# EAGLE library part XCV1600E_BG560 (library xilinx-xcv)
xcv1600e_bg560 edit this description Auto generated by make-symbol-device-package-bsdl.ulp Rev. 26 Source: xcv1600e_bg560.bsd
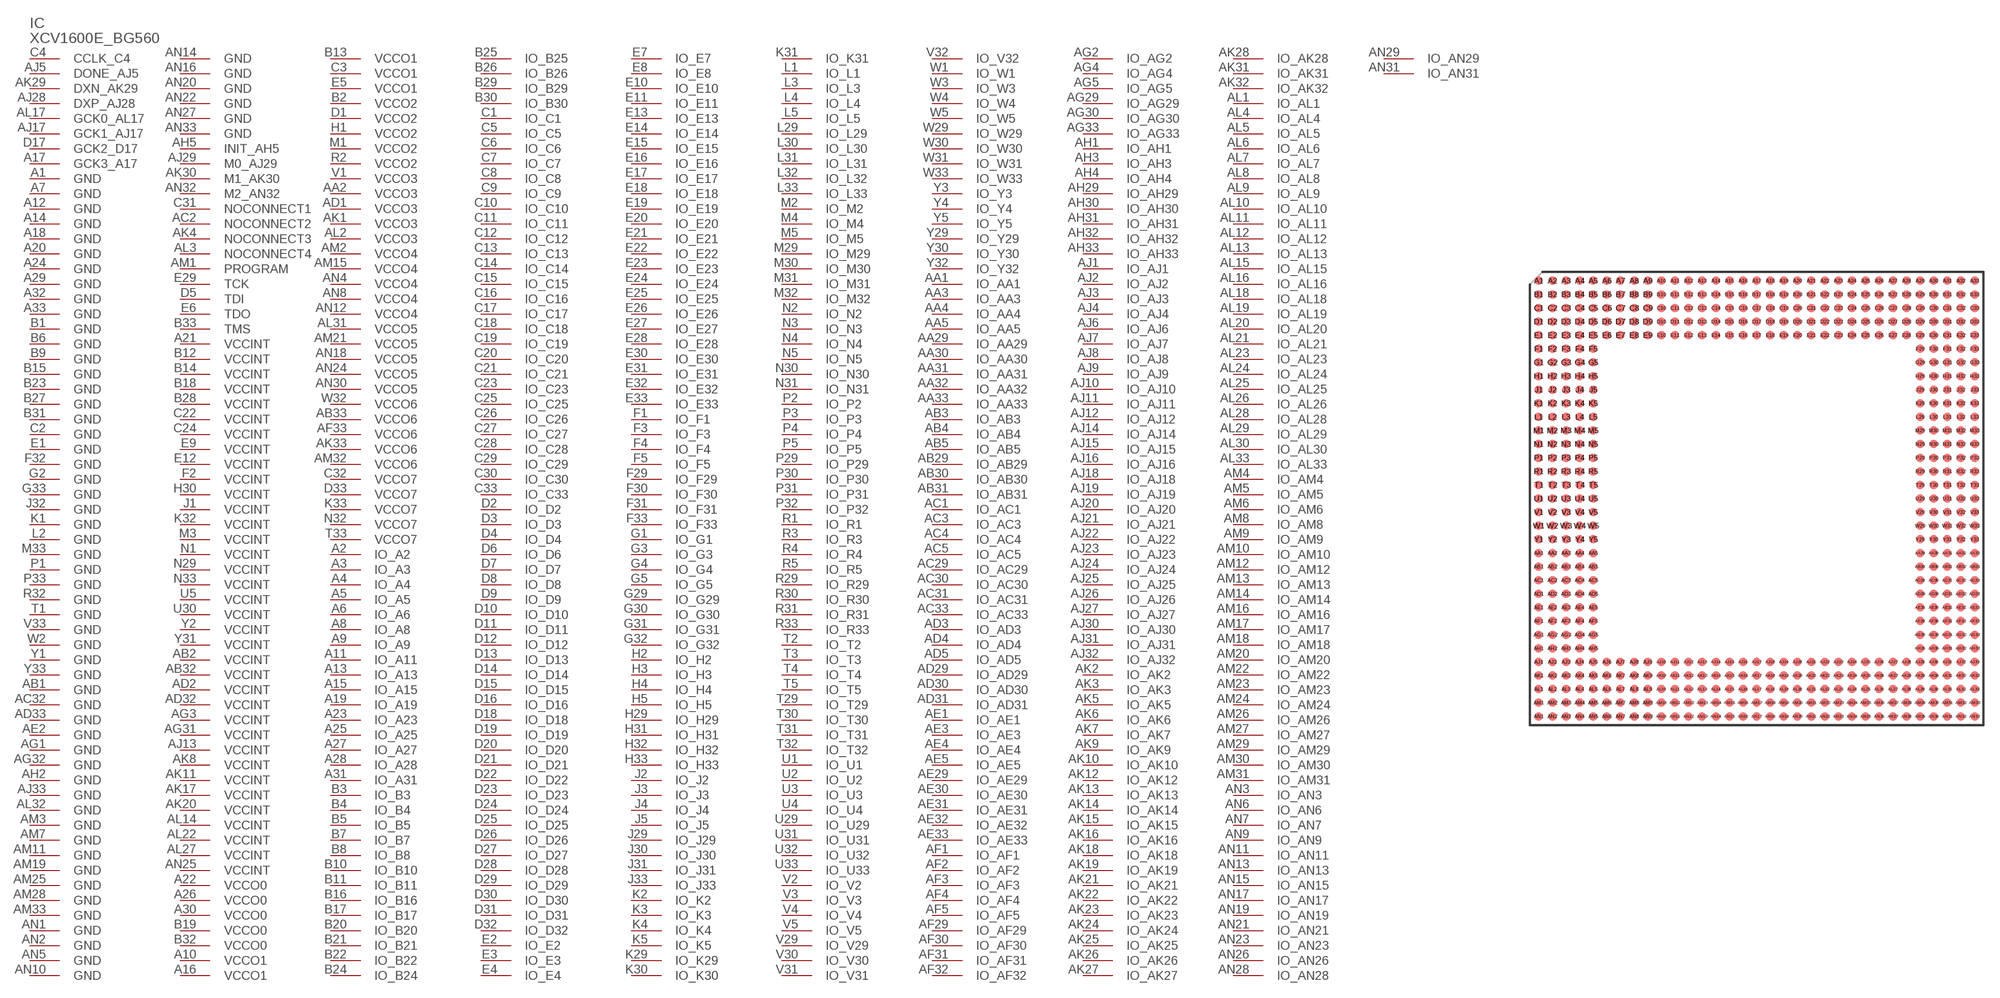
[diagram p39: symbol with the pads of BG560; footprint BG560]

Designator prefix IC

## XCV1600E_BG560 (OC_FARNELL: unknown; OC_NEWARK: unknown)  [BG560]
A1  GND  pwr
A2  IO_A2
A3  IO_A3
A4  IO_A4
A5  IO_A5
A6  IO_A6
A7  GND  pwr
A8  IO_A8
A9  IO_A9
A10  VCCO1  pwr
A11  IO_A11
A12  GND  pwr
A13  IO_A13
A14  GND  pwr
A15  IO_A15
A16  VCCO1  pwr
A17  GCK3_A17  in
A18  GND  pwr
A19  IO_A19
A20  GND  pwr
A21  VCCINT  pwr
A22  VCCO0  pwr
A23  IO_A23
A24  GND  pwr
A25  IO_A25
A26  VCCO0  pwr
A27  IO_A27
A28  IO_A28
A29  GND  pwr
A30  VCCO0  pwr
A31  IO_A31
A32  GND  pwr
A33  GND  pwr
AA1  IO_AA1
AA2  VCCO3  pwr
AA3  IO_AA3
AA4  IO_AA4
AA5  IO_AA5
AA29  IO_AA29
AA30  IO_AA30
AA31  IO_AA31
AA32  IO_AA32
AA33  IO_AA33
AB1  GND  pwr
AB2  VCCINT  pwr
AB3  IO_AB3
AB4  IO_AB4
AB5  IO_AB5
AB29  IO_AB29
AB30  IO_AB30
AB31  IO_AB31
AB32  VCCINT  pwr
AB33  VCCO6  pwr
AC1  IO_AC1
AC2  NOCONNECT2  pas
AC3  IO_AC3
AC4  IO_AC4
AC5  IO_AC5
AC29  IO_AC29
AC30  IO_AC30
AC31  IO_AC31
AC32  GND  pwr
AC33  IO_AC33
AD1  VCCO3  pwr
AD2  VCCINT  pwr
AD3  IO_AD3
AD4  IO_AD4
AD5  IO_AD5
AD29  IO_AD29
AD30  IO_AD30
AD31  IO_AD31
AD32  VCCINT  pwr
AD33  GND  pwr
AE1  IO_AE1
AE2  GND  pwr
AE3  IO_AE3
AE4  IO_AE4
AE5  IO_AE5
AE29  IO_AE29
AE30  IO_AE30
AE31  IO_AE31
AE32  IO_AE32
AE33  IO_AE33
AF1  IO_AF1
AF2  IO_AF2
AF3  IO_AF3
AF4  IO_AF4
AF5  IO_AF5
AF29  IO_AF29
AF30  IO_AF30
AF31  IO_AF31
AF32  IO_AF32
AF33  VCCO6  pwr
AG1  GND  pwr
AG2  IO_AG2
AG3  VCCINT  pwr
AG4  IO_AG4
AG5  IO_AG5
AG29  IO_AG29
AG30  IO_AG30
AG31  VCCINT  pwr
AG32  GND  pwr
AG33  IO_AG33
AH1  IO_AH1
AH2  GND  pwr
AH3  IO_AH3
AH4  IO_AH4
AH5  INIT_AH5
AH29  IO_AH29
AH30  IO_AH30
AH31  IO_AH31
AH32  IO_AH32
AH33  IO_AH33
AJ1  IO_AJ1
AJ2  IO_AJ2
AJ3  IO_AJ3
AJ4  IO_AJ4
AJ5  DONE_AJ5
AJ6  IO_AJ6
AJ7  IO_AJ7
AJ8  IO_AJ8
AJ9  IO_AJ9
AJ10  IO_AJ10
AJ11  IO_AJ11
AJ12  IO_AJ12
AJ13  VCCINT  pwr
AJ14  IO_AJ14
AJ15  IO_AJ15
AJ16  IO_AJ16
AJ17  GCK1_AJ17  in
AJ18  IO_AJ18
AJ19  IO_AJ19
AJ20  IO_AJ20
AJ21  IO_AJ21
AJ22  IO_AJ22
AJ23  IO_AJ23
AJ24  IO_AJ24
AJ25  IO_AJ25
AJ26  IO_AJ26
AJ27  IO_AJ27
AJ28  DXP_AJ28  pas
AJ29  M0_AJ29  in
AJ30  IO_AJ30
AJ31  IO_AJ31
AJ32  IO_AJ32
AJ33  GND  pwr
AK1  VCCO3  pwr
AK2  IO_AK2
AK3  IO_AK3
AK4  NOCONNECT3  pas
AK5  IO_AK5
AK6  IO_AK6
AK7  IO_AK7
AK8  VCCINT  pwr
AK9  IO_AK9
AK10  IO_AK10
AK11  VCCINT  pwr
AK12  IO_AK12
AK13  IO_AK13
AK14  IO_AK14
AK15  IO_AK15
AK16  IO_AK16
AK17  VCCINT  pwr
AK18  IO_AK18
AK19  IO_AK19
AK20  VCCINT  pwr
AK21  IO_AK21
AK22  IO_AK22
AK23  IO_AK23
AK24  IO_AK24
AK25  IO_AK25
AK26  IO_AK26
AK27  IO_AK27
AK28  IO_AK28
AK29  DXN_AK29  pas
AK30  M1_AK30  in
AK31  IO_AK31
AK32  IO_AK32
AK33  VCCO6  pwr
AL1  IO_AL1
AL2  VCCO3  pwr
AL3  NOCONNECT4  pas
AL4  IO_AL4
AL5  IO_AL5
AL6  IO_AL6
AL7  IO_AL7
AL8  IO_AL8
AL9  IO_AL9
AL10  IO_AL10
AL11  IO_AL11
AL12  IO_AL12
AL13  IO_AL13
AL14  VCCINT  pwr
AL15  IO_AL15
AL16  IO_AL16
AL17  GCK0_AL17  in
AL18  IO_AL18
AL19  IO_AL19
AL20  IO_AL20
AL21  IO_AL21
AL22  VCCINT  pwr
AL23  IO_AL23
AL24  IO_AL24
AL25  IO_AL25
AL26  IO_AL26
AL27  VCCINT  pwr
AL28  IO_AL28
AL29  IO_AL29
AL30  IO_AL30
AL31  VCCO5  pwr
AL32  GND  pwr
AL33  IO_AL33
AM1  PROGRAM  in
AM2  VCCO4  pwr
AM3  GND  pwr
AM4  IO_AM4
AM5  IO_AM5
AM6  IO_AM6
AM7  GND  pwr
AM8  IO_AM8
AM9  IO_AM9
AM10  IO_AM10
AM11  GND  pwr
AM12  IO_AM12
AM13  IO_AM13
AM14  IO_AM14
AM15  VCCO4  pwr
AM16  IO_AM16
AM17  IO_AM17
AM18  IO_AM18
AM19  GND  pwr
AM20  IO_AM20
AM21  VCCO5  pwr
AM22  IO_AM22
AM23  IO_AM23
AM24  IO_AM24
AM25  GND  pwr
AM26  IO_AM26
AM27  IO_AM27
AM28  GND  pwr
AM29  IO_AM29
AM30  IO_AM30
AM31  IO_AM31
AM32  VCCO6  pwr
AM33  GND  pwr
AN1  GND  pwr
AN2  GND  pwr
AN3  IO_AN3
AN4  VCCO4  pwr
AN5  GND  pwr
AN6  IO_AN6
AN7  IO_AN7
AN8  VCCO4  pwr
AN9  IO_AN9
AN10  GND  pwr
AN11  IO_AN11
AN12  VCCO4  pwr
AN13  IO_AN13
AN14  GND  pwr
AN15  IO_AN15
AN16  GND  pwr
AN17  IO_AN17
AN18  VCCO5  pwr
AN19  IO_AN19
AN20  GND  pwr
AN21  IO_AN21
AN22  GND  pwr
AN23  IO_AN23
AN24  VCCO5  pwr
AN25  VCCINT  pwr
AN26  IO_AN26
AN27  GND  pwr
AN28  IO_AN28
AN29  IO_AN29
AN30  VCCO5  pwr
AN31  IO_AN31
AN32  M2_AN32  in
AN33  GND  pwr
B1  GND  pwr
B2  VCCO2  pwr
B3  IO_B3
B4  IO_B4
B5  IO_B5
B6  GND  pwr
B7  IO_B7
B8  IO_B8
B9  GND  pwr
B10  IO_B10
B11  IO_B11
B12  VCCINT  pwr
B13  VCCO1  pwr
B14  VCCINT  pwr
B15  GND  pwr
B16  IO_B16
B17  IO_B17
B18  VCCINT  pwr
B19  VCCO0  pwr
B20  IO_B20
B21  IO_B21
B22  IO_B22
B23  GND  pwr
B24  IO_B24
B25  IO_B25
B26  IO_B26
B27  GND  pwr
B28  VCCINT  pwr
B29  IO_B29
B30  IO_B30
B31  GND  pwr
B32  VCCO0  pwr
B33  TMS  in
C1  IO_C1
C2  GND  pwr
C3  VCCO1  pwr
C4  CCLK_C4
C5  IO_C5
C6  IO_C6
C7  IO_C7
C8  IO_C8
C9  IO_C9
C10  IO_C10
C11  IO_C11
C12  IO_C12
C13  IO_C13
C14  IO_C14
C15  IO_C15
C16  IO_C16
C17  IO_C17
C18  IO_C18
C19  IO_C19
C20  IO_C20
C21  IO_C21
C22  VCCINT  pwr
C23  IO_C23
C24  VCCINT  pwr
C25  IO_C25
C26  IO_C26
C27  IO_C27
C28  IO_C28
C29  IO_C29
C30  IO_C30
C31  NOCONNECT1  pas
C32  VCCO7  pwr
C33  IO_C33
D1  VCCO2  pwr
D2  IO_D2
D3  IO_D3
D4  IO_D4
D5  TDI  in
D6  IO_D6
D7  IO_D7
D8  IO_D8
D9  IO_D9
D10  IO_D10
D11  IO_D11
D12  IO_D12
D13  IO_D13
D14  IO_D14
D15  IO_D15
D16  IO_D16
D17  GCK2_D17  in
D18  IO_D18
D19  IO_D19
D20  IO_D20
D21  IO_D21
D22  IO_D22
D23  IO_D23
D24  IO_D24
D25  IO_D25
D26  IO_D26
D27  IO_D27
D28  IO_D28
D29  IO_D29
D30  IO_D30
D31  IO_D31
D32  IO_D32
D33  VCCO7  pwr
E1  GND  pwr
E2  IO_E2
E3  IO_E3
E4  IO_E4
E5  VCCO1  pwr
E6  TDO  out
E7  IO_E7
E8  IO_E8
E9  VCCINT  pwr
E10  IO_E10
E11  IO_E11
E12  VCCINT  pwr
E13  IO_E13
E14  IO_E14
E15  IO_E15
E16  IO_E16
E17  IO_E17
E18  IO_E18
E19  IO_E19
E20  IO_E20
E21  IO_E21
E22  IO_E22
E23  IO_E23
E24  IO_E24
E25  IO_E25
E26  IO_E26
E27  IO_E27
E28  IO_E28
E29  TCK  in
E30  IO_E30
E31  IO_E31
E32  IO_E32
E33  IO_E33
F1  IO_F1
F2  VCCINT  pwr
F3  IO_F3
F4  IO_F4
F5  IO_F5
F29  IO_F29
F30  IO_F30
F31  IO_F31
F32  GND  pwr
F33  IO_F33
G1  IO_G1
G2  GND  pwr
G3  IO_G3
G4  IO_G4
G5  IO_G5
G29  IO_G29
G30  IO_G30
G31  IO_G31
G32  IO_G32
G33  GND  pwr
H1  VCCO2  pwr
H2  IO_H2
H3  IO_H3
H4  IO_H4
H5  IO_H5
H29  IO_H29
H30  VCCINT  pwr
H31  IO_H31
H32  IO_H32
H33  IO_H33
J1  VCCINT  pwr
J2  IO_J2
J3  IO_J3
J4  IO_J4
J5  IO_J5
J29  IO_J29
J30  IO_J30
J31  IO_J31
J32  GND  pwr
J33  IO_J33
K1  GND  pwr
K2  IO_K2
K3  IO_K3
K4  IO_K4
K5  IO_K5
K29  IO_K29
K30  IO_K30
K31  IO_K31
K32  VCCINT  pwr
K33  VCCO7  pwr
L1  IO_L1
L2  GND  pwr
L3  IO_L3
L4  IO_L4
L5  IO_L5
L29  IO_L29
L30  IO_L30
L31  IO_L31
L32  IO_L32
L33  IO_L33
M1  VCCO2  pwr
M2  IO_M2
M3  VCCINT  pwr
M4  IO_M4
M5  IO_M5
M29  IO_M29
M30  IO_M30
M31  IO_M31
M32  IO_M32
M33  GND  pwr
N1  VCCINT  pwr
N2  IO_N2
N3  IO_N3
N4  IO_N4
N5  IO_N5
N29  VCCINT  pwr
N30  IO_N30
N31  IO_N31
N32  VCCO7  pwr
N33  VCCINT  pwr
P1  GND  pwr
P2  IO_P2
P3  IO_P3
P4  IO_P4
P5  IO_P5
P29  IO_P29
P30  IO_P30
P31  IO_P31
P32  IO_P32
P33  GND  pwr
R1  IO_R1
R2  VCCO2  pwr
R3  IO_R3
R4  IO_R4
R5  IO_R5
R29  IO_R29
R30  IO_R30
R31  IO_R31
R32  GND  pwr
R33  IO_R33
T1  GND  pwr
T2  IO_T2
T3  IO_T3
T4  IO_T4
T5  IO_T5
T29  IO_T29
T30  IO_T30
T31  IO_T31
T32  IO_T32
T33  VCCO7  pwr
U1  IO_U1
U2  IO_U2
U3  IO_U3
U4  IO_U4
U5  VCCINT  pwr
U29  IO_U29
U30  VCCINT  pwr
U31  IO_U31
U32  IO_U32
U33  IO_U33
V1  VCCO3  pwr
V2  IO_V2
V3  IO_V3
V4  IO_V4
V5  IO_V5
V29  IO_V29
V30  IO_V30
V31  IO_V31
V32  IO_V32
V33  GND  pwr
W1  IO_W1
W2  GND  pwr
W3  IO_W3
W4  IO_W4
W5  IO_W5
W29  IO_W29
W30  IO_W30
W31  IO_W31
W32  VCCO6  pwr
W33  IO_W33
Y1  GND  pwr
Y2  VCCINT  pwr
Y3  IO_Y3
Y4  IO_Y4
Y5  IO_Y5
Y29  IO_Y29
Y30  IO_Y30
Y31  VCCINT  pwr
Y32  IO_Y32
Y33  GND  pwr

## Footprint BG560 (pad centres in mm)
Metal BGA (BG560) Auto generated by make-symbol-device-package-bsdl.ulp Rev. 26 Source: xcv1000_bg560_1532.bsd; bg560.pdf
smd 0.8 x 0.8: A1 -20.32,20.32; A2 -19.05,20.32; A3 -17.78,20.32; A4 -16.51,20.32; A5 -15.24,20.32; A6 -13.97,20.32; A7 -12.7,20.32; A8 -11.43,20.32; A9 -10.16,20.32; A10 -8.89,20.32; A11 -7.62,20.32; A12 -6.35,20.32; A13 -5.08,20.32; A14 -3.81,20.32; A15 -2.54,20.32; A16 -1.27,20.32; A17 0,20.32; A18 1.27,20.32; A19 2.54,20.32; A20 3.81,20.32; A21 5.08,20.32; A22 6.35,20.32; A23 7.62,20.32; A24 8.89,20.32; A25 10.16,20.32; A26 11.43,20.32; A27 12.7,20.32; A28 13.97,20.32; A29 15.24,20.32; A30 16.51,20.32; A31 17.78,20.32; A32 19.05,20.32; A33 20.32,20.32; AA1 -20.32,-5.08; AA2 -19.05,-5.08; AA3 -17.78,-5.08; AA4 -16.51,-5.08; AA5 -15.24,-5.08; AA29 15.24,-5.08; AA30 16.51,-5.08; AA31 17.78,-5.08; AA32 19.05,-5.08; AA33 20.32,-5.08; AB1 -20.32,-6.35; AB2 -19.05,-6.35; AB3 -17.78,-6.35; AB4 -16.51,-6.35; AB5 -15.24,-6.35; AB29 15.24,-6.35; AB30 16.51,-6.35; AB31 17.78,-6.35; AB32 19.05,-6.35; AB33 20.32,-6.35; AC1 -20.32,-7.62; AC2 -19.05,-7.62; AC3 -17.78,-7.62; AC4 -16.51,-7.62; AC5 -15.24,-7.62; AC29 15.24,-7.62; AC30 16.51,-7.62; AC31 17.78,-7.62; AC32 19.05,-7.62; AC33 20.32,-7.62; AD1 -20.32,-8.89; AD2 -19.05,-8.89; AD3 -17.78,-8.89; AD4 -16.51,-8.89; AD5 -15.24,-8.89; AD29 15.24,-8.89; AD30 16.51,-8.89; AD31 17.78,-8.89; AD32 19.05,-8.89; AD33 20.32,-8.89; AE1 -20.32,-10.16; AE2 -19.05,-10.16; AE3 -17.78,-10.16; AE4 -16.51,-10.16; AE5 -15.24,-10.16; AE29 15.24,-10.16; AE30 16.51,-10.16; AE31 17.78,-10.16; AE32 19.05,-10.16; AE33 20.32,-10.16; AF1 -20.32,-11.43; AF2 -19.05,-11.43; AF3 -17.78,-11.43; AF4 -16.51,-11.43; AF5 -15.24,-11.43; AF29 15.24,-11.43; AF30 16.51,-11.43; AF31 17.78,-11.43; AF32 19.05,-11.43; AF33 20.32,-11.43; AG1 -20.32,-12.7; AG2 -19.05,-12.7; AG3 -17.78,-12.7; AG4 -16.51,-12.7; AG5 -15.24,-12.7; AG29 15.24,-12.7; AG30 16.51,-12.7; AG31 17.78,-12.7; AG32 19.05,-12.7; AG33 20.32,-12.7; AH1 -20.32,-13.97; AH2 -19.05,-13.97; AH3 -17.78,-13.97; AH4 -16.51,-13.97; AH5 -15.24,-13.97; AH29 15.24,-13.97; AH30 16.51,-13.97; AH31 17.78,-13.97; AH32 19.05,-13.97; AH33 20.32,-13.97; AJ1 -20.32,-15.24; AJ2 -19.05,-15.24; AJ3 -17.78,-15.24; AJ4 -16.51,-15.24; AJ5 -15.24,-15.24; AJ6 -13.97,-15.24; AJ7 -12.7,-15.24; AJ8 -11.43,-15.24; AJ9 -10.16,-15.24; AJ10 -8.89,-15.24; AJ11 -7.62,-15.24; AJ12 -6.35,-15.24; AJ13 -5.08,-15.24; AJ14 -3.81,-15.24; AJ15 -2.54,-15.24; AJ16 -1.27,-15.24; AJ17 0,-15.24; AJ18 1.27,-15.24; AJ19 2.54,-15.24; AJ20 3.81,-15.24; AJ21 5.08,-15.24; AJ22 6.35,-15.24; AJ23 7.62,-15.24; AJ24 8.89,-15.24; AJ25 10.16,-15.24; AJ26 11.43,-15.24; AJ27 12.7,-15.24; AJ28 13.97,-15.24; AJ29 15.24,-15.24; AJ30 16.51,-15.24; AJ31 17.78,-15.24; AJ32 19.05,-15.24; AJ33 20.32,-15.24; AK1 -20.32,-16.51; AK2 -19.05,-16.51; AK3 -17.78,-16.51; AK4 -16.51,-16.51; AK5 -15.24,-16.51; AK6 -13.97,-16.51; AK7 -12.7,-16.51; AK8 -11.43,-16.51; AK9 -10.16,-16.51; AK10 -8.89,-16.51; AK11 -7.62,-16.51; AK12 -6.35,-16.51; AK13 -5.08,-16.51; AK14 -3.81,-16.51; AK15 -2.54,-16.51; AK16 -1.27,-16.51; AK17 0,-16.51; AK18 1.27,-16.51; AK19 2.54,-16.51; AK20 3.81,-16.51; AK21 5.08,-16.51; AK22 6.35,-16.51; AK23 7.62,-16.51; AK24 8.89,-16.51; AK25 10.16,-16.51; AK26 11.43,-16.51; AK27 12.7,-16.51; AK28 13.97,-16.51; AK29 15.24,-16.51; AK30 16.51,-16.51; AK31 17.78,-16.51; AK32 19.05,-16.51; AK33 20.32,-16.51; AL1 -20.32,-17.78; AL2 -19.05,-17.78; AL3 -17.78,-17.78; AL4 -16.51,-17.78; AL5 -15.24,-17.78; AL6 -13.97,-17.78; AL7 -12.7,-17.78; AL8 -11.43,-17.78; AL9 -10.16,-17.78; AL10 -8.89,-17.78; AL11 -7.62,-17.78; AL12 -6.35,-17.78; AL13 -5.08,-17.78; AL14 -3.81,-17.78; AL15 -2.54,-17.78; AL16 -1.27,-17.78; AL17 0,-17.78; AL18 1.27,-17.78; AL19 2.54,-17.78; AL20 3.81,-17.78; AL21 5.08,-17.78; AL22 6.35,-17.78; AL23 7.62,-17.78; AL24 8.89,-17.78; AL25 10.16,-17.78; AL26 11.43,-17.78; AL27 12.7,-17.78; AL28 13.97,-17.78; AL29 15.24,-17.78; AL30 16.51,-17.78; AL31 17.78,-17.78; AL32 19.05,-17.78; AL33 20.32,-17.78; AM1 -20.32,-19.05; AM2 -19.05,-19.05; AM3 -17.78,-19.05; AM4 -16.51,-19.05; AM5 -15.24,-19.05; AM6 -13.97,-19.05; AM7 -12.7,-19.05; AM8 -11.43,-19.05; AM9 -10.16,-19.05; AM10 -8.89,-19.05; AM11 -7.62,-19.05; AM12 -6.35,-19.05; AM13 -5.08,-19.05; AM14 -3.81,-19.05; AM15 -2.54,-19.05; AM16 -1.27,-19.05; AM17 0,-19.05; AM18 1.27,-19.05; AM19 2.54,-19.05; AM20 3.81,-19.05; AM21 5.08,-19.05; AM22 6.35,-19.05; AM23 7.62,-19.05; AM24 8.89,-19.05; AM25 10.16,-19.05; AM26 11.43,-19.05; AM27 12.7,-19.05; AM28 13.97,-19.05; AM29 15.24,-19.05; AM30 16.51,-19.05; AM31 17.78,-19.05; AM32 19.05,-19.05; AM33 20.32,-19.05; AN1 -20.32,-20.32; AN2 -19.05,-20.32; AN3 -17.78,-20.32; AN4 -16.51,-20.32; AN5 -15.24,-20.32; AN6 -13.97,-20.32; AN7 -12.7,-20.32; AN8 -11.43,-20.32; AN9 -10.16,-20.32; AN10 -8.89,-20.32; AN11 -7.62,-20.32; AN12 -6.35,-20.32; AN13 -5.08,-20.32; AN14 -3.81,-20.32; AN15 -2.54,-20.32; AN16 -1.27,-20.32; AN17 0,-20.32; AN18 1.27,-20.32; AN19 2.54,-20.32; AN20 3.81,-20.32; AN21 5.08,-20.32; AN22 6.35,-20.32; AN23 7.62,-20.32; AN24 8.89,-20.32; AN25 10.16,-20.32; AN26 11.43,-20.32; AN27 12.7,-20.32; AN28 13.97,-20.32; AN29 15.24,-20.32; AN30 16.51,-20.32; AN31 17.78,-20.32; AN32 19.05,-20.32; AN33 20.32,-20.32; B1 -20.32,19.05; B2 -19.05,19.05; B3 -17.78,19.05; B4 -16.51,19.05; B5 -15.24,19.05; B6 -13.97,19.05; B7 -12.7,19.05; B8 -11.43,19.05; B9 -10.16,19.05; B10 -8.89,19.05; B11 -7.62,19.05; B12 -6.35,19.05; B13 -5.08,19.05; B14 -3.81,19.05; B15 -2.54,19.05; B16 -1.27,19.05; B17 0,19.05; B18 1.27,19.05; B19 2.54,19.05; B20 3.81,19.05; B21 5.08,19.05; B22 6.35,19.05; B23 7.62,19.05; B24 8.89,19.05; B25 10.16,19.05; B26 11.43,19.05; B27 12.7,19.05; B28 13.97,19.05; B29 15.24,19.05; B30 16.51,19.05; B31 17.78,19.05; B32 19.05,19.05; B33 20.32,19.05; C1 -20.32,17.78; C2 -19.05,17.78; C3 -17.78,17.78; C4 -16.51,17.78; C5 -15.24,17.78; C6 -13.97,17.78; C7 -12.7,17.78; C8 -11.43,17.78; C9 -10.16,17.78; C10 -8.89,17.78; C11 -7.62,17.78; C12 -6.35,17.78; C13 -5.08,17.78; C14 -3.81,17.78; C15 -2.54,17.78; C16 -1.27,17.78; C17 0,17.78; C18 1.27,17.78; C19 2.54,17.78; C20 3.81,17.78; C21 5.08,17.78; C22 6.35,17.78; C23 7.62,17.78; C24 8.89,17.78; C25 10.16,17.78; C26 11.43,17.78; C27 12.7,17.78; C28 13.97,17.78; C29 15.24,17.78; C30 16.51,17.78; C31 17.78,17.78; C32 19.05,17.78; C33 20.32,17.78; D1 -20.32,16.51; D2 -19.05,16.51; D3 -17.78,16.51; D4 -16.51,16.51; D5 -15.24,16.51; D6 -13.97,16.51; D7 -12.7,16.51; D8 -11.43,16.51; D9 -10.16,16.51; D10 -8.89,16.51; D11 -7.62,16.51; D12 -6.35,16.51; D13 -5.08,16.51; D14 -3.81,16.51; D15 -2.54,16.51; D16 -1.27,16.51; D17 0,16.51; D18 1.27,16.51; D19 2.54,16.51; D20 3.81,16.51; D21 5.08,16.51; D22 6.35,16.51; D23 7.62,16.51; D24 8.89,16.51; D25 10.16,16.51; D26 11.43,16.51; D27 12.7,16.51; D28 13.97,16.51; D29 15.24,16.51; D30 16.51,16.51; D31 17.78,16.51; D32 19.05,16.51; D33 20.32,16.51; E1 -20.32,15.24; E2 -19.05,15.24; E3 -17.78,15.24; E4 -16.51,15.24; E5 -15.24,15.24; E6 -13.97,15.24; E7 -12.7,15.24; E8 -11.43,15.24; E9 -10.16,15.24; E10 -8.89,15.24; E11 -7.62,15.24; E12 -6.35,15.24; E13 -5.08,15.24; E14 -3.81,15.24; E15 -2.54,15.24; E16 -1.27,15.24; E17 0,15.24; E18 1.27,15.24; E19 2.54,15.24; E20 3.81,15.24; E21 5.08,15.24; E22 6.35,15.24; E23 7.62,15.24; E24 8.89,15.24; E25 10.16,15.24; E26 11.43,15.24; E27 12.7,15.24; E28 13.97,15.24; E29 15.24,15.24; E30 16.51,15.24; E31 17.78,15.24; E32 19.05,15.24; E33 20.32,15.24; F1 -20.32,13.97; F2 -19.05,13.97; F3 -17.78,13.97; F4 -16.51,13.97; F5 -15.24,13.97; F29 15.24,13.97; F30 16.51,13.97; F31 17.78,13.97; F32 19.05,13.97; F33 20.32,13.97; G1 -20.32,12.7; G2 -19.05,12.7; G3 -17.78,12.7; G4 -16.51,12.7; G5 -15.24,12.7; G29 15.24,12.7; G30 16.51,12.7; G31 17.78,12.7; G32 19.05,12.7; G33 20.32,12.7; H1 -20.32,11.43; H2 -19.05,11.43; H3 -17.78,11.43; H4 -16.51,11.43; H5 -15.24,11.43; H29 15.24,11.43; H30 16.51,11.43; H31 17.78,11.43; H32 19.05,11.43; H33 20.32,11.43; J1 -20.32,10.16; J2 -19.05,10.16; J3 -17.78,10.16; J4 -16.51,10.16; J5 -15.24,10.16; J29 15.24,10.16; J30 16.51,10.16; J31 17.78,10.16; J32 19.05,10.16; J33 20.32,10.16; K1 -20.32,8.89; K2 -19.05,8.89; K3 -17.78,8.89; K4 -16.51,8.89; K5 -15.24,8.89; K29 15.24,8.89; K30 16.51,8.89; K31 17.78,8.89; K32 19.05,8.89; K33 20.32,8.89; L1 -20.32,7.62; L2 -19.05,7.62; L3 -17.78,7.62; L4 -16.51,7.62; L5 -15.24,7.62; L29 15.24,7.62; L30 16.51,7.62; L31 17.78,7.62; L32 19.05,7.62; L33 20.32,7.62; M1 -20.32,6.35; M2 -19.05,6.35; M3 -17.78,6.35; M4 -16.51,6.35; M5 -15.24,6.35; M29 15.24,6.35; M30 16.51,6.35; M31 17.78,6.35; M32 19.05,6.35; M33 20.32,6.35; N1 -20.32,5.08; N2 -19.05,5.08; N3 -17.78,5.08; N4 -16.51,5.08; N5 -15.24,5.08; N29 15.24,5.08; N30 16.51,5.08; N31 17.78,5.08; N32 19.05,5.08; N33 20.32,5.08; P1 -20.32,3.81; P2 -19.05,3.81; P3 -17.78,3.81; P4 -16.51,3.81; P5 -15.24,3.81; P29 15.24,3.81; P30 16.51,3.81; P31 17.78,3.81; P32 19.05,3.81; P33 20.32,3.81; R1 -20.32,2.54; R2 -19.05,2.54; R3 -17.78,2.54; R4 -16.51,2.54; R5 -15.24,2.54; R29 15.24,2.54; R30 16.51,2.54; R31 17.78,2.54; R32 19.05,2.54; R33 20.32,2.54; T1 -20.32,1.27; T2 -19.05,1.27; T3 -17.78,1.27; T4 -16.51,1.27; T5 -15.24,1.27; T29 15.24,1.27; T30 16.51,1.27; T31 17.78,1.27; T32 19.05,1.27; T33 20.32,1.27; U1 -20.32,0; U2 -19.05,0; U3 -17.78,0; U4 -16.51,0; U5 -15.24,0; U29 15.24,0; U30 16.51,0; U31 17.78,0; U32 19.05,0; U33 20.32,0; V1 -20.32,-1.27; V2 -19.05,-1.27; V3 -17.78,-1.27; V4 -16.51,-1.27; V5 -15.24,-1.27; V29 15.24,-1.27; V30 16.51,-1.27; V31 17.78,-1.27; V32 19.05,-1.27; V33 20.32,-1.27; W1 -20.32,-2.54; W2 -19.05,-2.54; W3 -17.78,-2.54; W4 -16.51,-2.54; W5 -15.24,-2.54; W29 15.24,-2.54; W30 16.51,-2.54; W31 17.78,-2.54; W32 19.05,-2.54; W33 20.32,-2.54; Y1 -20.32,-3.81; Y2 -19.05,-3.81; Y3 -17.78,-3.81; Y4 -16.51,-3.81; Y5 -15.24,-3.81; Y29 15.24,-3.81; Y30 16.51,-3.81; Y31 17.78,-3.81; Y32 19.05,-3.81; Y33 20.32,-3.81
